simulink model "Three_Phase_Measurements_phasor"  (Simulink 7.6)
settings: Solver=ode23tb  StartTime=0.0  StopTime=0.05  RelTol=1e-3
StopFcn:
  | if 0
  | close all, clc
  | load amplitude_phase.mat
  | plotyy(x(1,:),x(2,:), x(1,:),x(3,:))
  | grid
  | title('Amplitude et Phase de la tension sur la phase A')
  | xlabel('temps')
  | 
  | figure
  | load tension_ValEfficace.mat
  | plotyy(z(1,:),z(2,:))
  | grid
  | title('Tension et valeur éfficace de la phase A')
  | xlabel('temps')
  | end
libraries: powerlib x10

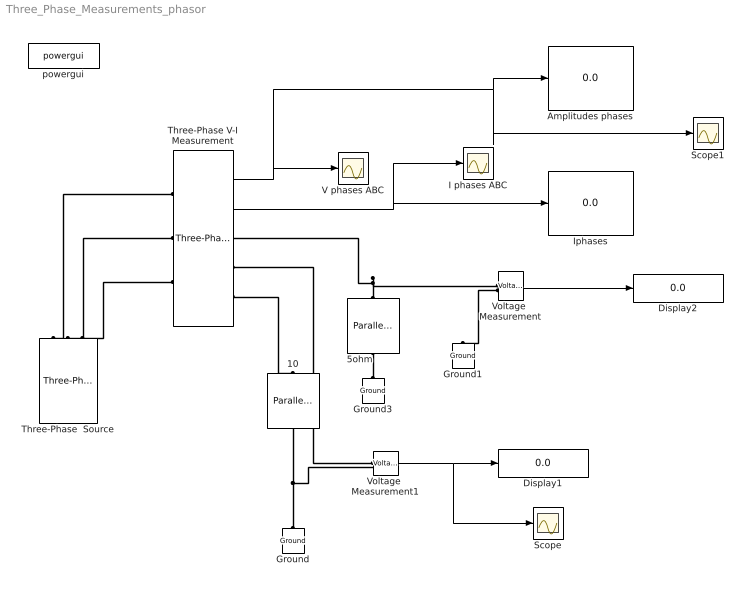
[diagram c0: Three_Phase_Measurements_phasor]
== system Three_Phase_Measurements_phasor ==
  10 : powerlib/Elements/Parallel RLC Branch  DialogController=POWERSYS.PowerSysDialog  PhysicalDomain=powersysdomain  SubClassName=unknown  LeftPortType=p1  RightPortType=p1  LConnTagsString=a  RConnTagsString=__new0  BranchType=R  Resistance=10  Inductance=1e-3  SetiL0=off  InitialCurrent=0  Capacitance=1e-6  Setx0=off  InitialVoltage=0  Measurements=None
  5ohm : powerlib/Elements/Parallel RLC Branch  DialogController=POWERSYS.PowerSysDialog  PhysicalDomain=powersysdomain  SubClassName=unknown  LeftPortType=p1  RightPortType=p1  LConnTagsString=a  RConnTagsString=__new0  BranchType=R  Resistance=5  Inductance=1e-3  SetiL0=off  InitialCurrent=0  Capacitance=1e-6  Setx0=off  InitialVoltage=0  Measurements=None
  Amplitudes phases : Display
  Display1 : Display
  Display2 : Display
  Ground : powerlib/Elements/Ground  DialogController=POWERSYS.PowerSysDialog  PhysicalDomain=powersysdomain  SubClassName=unknown  LeftPortType=p1  RightPortType=p1  LConnTagsString=a
  Ground1 : powerlib/Elements/Ground  DialogController=POWERSYS.PowerSysDialog  PhysicalDomain=powersysdomain  SubClassName=unknown  LeftPortType=p1  RightPortType=p1  LConnTagsString=a
  Ground3 : powerlib/Elements/Ground  DialogController=POWERSYS.PowerSysDialog  PhysicalDomain=powersysdomain  SubClassName=unknown  LeftPortType=p1  RightPortType=p1  LConnTagsString=a
  I phases ABC : Scope
  Iphases : Display
  Scope : Scope
  Scope1 : Scope
  Three-Phase V-I Measurement : powerlib/Measurements/Three-Phase V-I Measurement  DialogController=POWERSYS.PowerSysDialog  SystemSampleTime=-1  VoltageMeasurement=phase-to-ground  SetLabelV=off  LabelV=Vabc  Vpu=off  VpuLL=off  CurrentMeasurement=yes  SetLabelI=off  LabelI=Iabc  Ipu=off  Pbase=100e6  Vbase=500e3  OutputType=Magnitude  PhasorSimulation=on  PSBequivalent=0
  Three-Phase  Source : powerlib/Electrical Sources/Three-Phase Source  DialogController=POWERSYS.PowerSysDialog  SystemSampleTime=-1  Voltage=220*sqrt(3)  PhaseAngle=0  Frequency=60  InternalConnection=Yg  SpecifyImpedance=off  Resistance=1  Inductance=10e-3  ShortCircuitLevel=100e6  BaseVoltage=25e3  XRratio=7
  V phases ABC : Scope
  Voltage  Measurement : powerlib/Measurements/Voltage Measurement  DialogController=POWERSYS.PowerSysDialog  SystemSampleTime=-1  PhasorSimulation=on  OutputType=Magnitude  PSBequivalent=0
  Voltage  Measurement1 : powerlib/Measurements/Voltage Measurement  DialogController=POWERSYS.PowerSysDialog  SystemSampleTime=-1  PhasorSimulation=on  OutputType=Magnitude  PSBequivalent=0
  powergui : powerlib/powergui  SystemSampleTime=-1  SimulationMode=Phasor  SampleTime=1e-5  frequency=60  SPID=on  DisableSnubberDevices=off  DisableRonSwitches=off  DisableVfSwitches=off  SwTol=0  Interpol=off  frequencyindice=60  echomessages=off  HookPort=off  DisplayEquations=off  FunctionMessages=off  EnableUseOfTLC=off  x0status=blocks  RestoreLinks=warning  ResistiveCurrentMeasurement=off  Frange=[0:2:500]  Ylog=off  Xlog=on  ShowGrid=off  save=off  variable=ZData  structure=ScopeData1  ZoomFFT=off  StartTime=0.0  cycles=1  DisplayStyle=1  fundamental=10  FreqAxis=off  MaxFrequency=100  frequencyindicesteady=60  RmsSteady=1  display=off  Ts=0  methode=off
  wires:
  Three-Phase V-I Measurement/1 -> V phases ABC/1, Amplitudes phases/1, Scope1/1
  Three-Phase V-I Measurement/2 -> Iphases/1, I phases ABC/1
  Voltage  Measurement/1 -> Display2/1
  Voltage  Measurement1/1 -> Display1/1, Scope/1
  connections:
  Three-Phase V-I Measurement/LConn3 -- Three-Phase  Source/RConn3
  Three-Phase V-I Measurement/LConn2 -- Three-Phase  Source/RConn2
  Three-Phase V-I Measurement/RConn3 -- 10/RConn1
  5ohm/LConn1 -- Ground3/LConn1
  Three-Phase V-I Measurement/LConn1 -- Three-Phase  Source/RConn1
  5ohm/RConn1 -- Three-Phase V-I Measurement/RConn1 -- Voltage  Measurement/LConn1
  Voltage  Measurement/LConn2 -- Ground1/LConn1
  Ground/LConn1 -- Voltage  Measurement1/LConn2 -- 10/LConn1
  Three-Phase V-I Measurement/RConn2 -- Voltage  Measurement1/LConn1
